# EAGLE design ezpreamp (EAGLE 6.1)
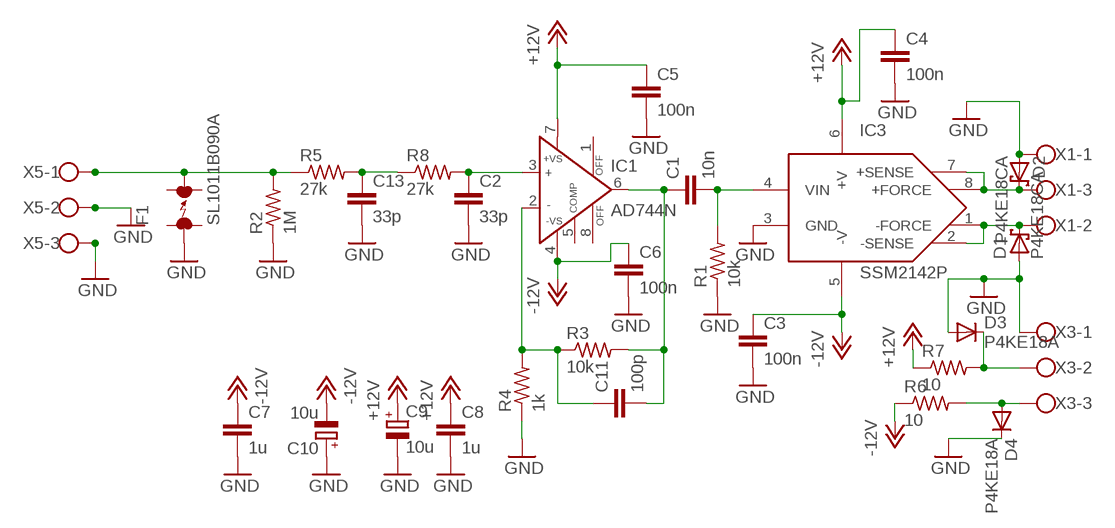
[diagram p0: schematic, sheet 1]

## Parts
C1  10n  C5/3  [C5B3]
C2  33p  C5/3  [C5B3]
C3  100n  C5/2.5  [C5B2.5]
C4  100n  C5/2.5  [C5B2.5]
C5  100n  C5/2.5  [C5B2.5]
C6  100n  C5/2.5  [C5B2.5]
C7  1u  C5/2.5  [C5B2.5]
C8  1u  C5/2.5  [C5B2.5]
C9  10u  CPOL-EUE5-10.5  [E5-10,5]
C10  10u  CPOL-EUE5-10.5  [E5-10,5]
C11  100p  C5/3  [C5B3]
C13  33p  C5/3  [C5B3]
D1  P4KE18CA  P4KEXX  [DO41-10]
D2  P4KE18CA  P4KEXX  [DO41-10]
D3  P4KE18A  1N4004  [DO41-10]
D4  P4KE18A  1N4004  [DO41-10]
F1  SL1011B090A  ARRESTER  [EPCOS_N81]
IC1  AD744N  [DIL08]
IC3  SSM2142P  [N-8]
R1  10k  R-US_0207/10  [0207/10]
R2  1M  R-US_0207/10  [0207/10]
R3  10k  R-US_0207/10  [0207/10]
R4  1k  R-US_0207/10  [0207/10]
R5  27k  R-US_0207/10  [0207/10]
R6  10  R-US_0207/10  [0207/10]
R7  10  R-US_0207/10  [0207/10]
R8  27k  R-US_0207/10  [0207/10]
X1  W237-103  [W237-103]
X3  W237-103  [W237-103]
X5  W237-103  [W237-103]

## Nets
+12V: C4.1 C5.1 C8.1 C9.+ IC1.7(+VS) IC3.6(+V) R7.1
-12V: C3.1 C6.1 C7.1 C10.- IC1.4(-VS) IC3.5(-V) R6.1
GND: C2.2 C3.2 C4.2 C5.2 C6.2 C7.2 C8.2 C9.- C10.+ C13.2 D1.A D2.A D3.A D4.C F1.1 IC3.3(GND) R1.1 R2.1 R4.1 X1.1 X3.1 X5.2 X5.3
N$1: C2.1 IC1.3(IN+) R8.2
N$2: C13.1 R5.2 R8.1
N$3: C1.2 IC3.4(VIN) R1.2
N$4: C1.1 C11.2 IC1.6(OUT) R3.2
N$5: F1.2 R2.2 R5.1 X5.1
N$6: D2.C IC3.7(+SENSE) IC3.8(+FORCE) X1.3
N$7: D1.C IC3.1(-FORCE) IC3.2(-SENSE) X1.2
N$8: C11.1 IC1.2(IN-) R3.1 R4.2
N$13: D4.A R6.2 X3.3
N$14: D3.C R7.2 X3.2
Unconnected: IC1.1(OFF) IC1.5(COMP) IC1.8(OFF)

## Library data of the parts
C1-C8 C11 C13 = capacitor-wima:C: CAPACITOR
C9 C10 = resistor:CPOL-EU: POLARIZED CAPACITOR, European symbol
D1 D2 = diode:P4KEXX: DIODE
D3 D4 = diode:1N4004: DIODE
F1 = discrete:ARRESTER: GASENTLADUNGSABLEITER 90V 10KA
IC1 = analog-devices:AD744: Precision, 500 ns Settling BiFET Op Amp Source: http://www.analog.com/static/imported-files/data_sheets/AD744.pdf; MF: ALTERA CORPORATION; MPN: AD744JNZ; OC_FARNELL: 1438362; OC_NEWARK: 59K4810
IC3 = JBB:SSM2142P
R1-R8 = rcl:R-US_: RESISTOR, American symbol
X1 X3 X5 = con-wago-500:W237-103: WAGO SCREW CLAMP; MPN: 237-103; OC_FARNELL: unknown; OC_NEWARK: 18M7116

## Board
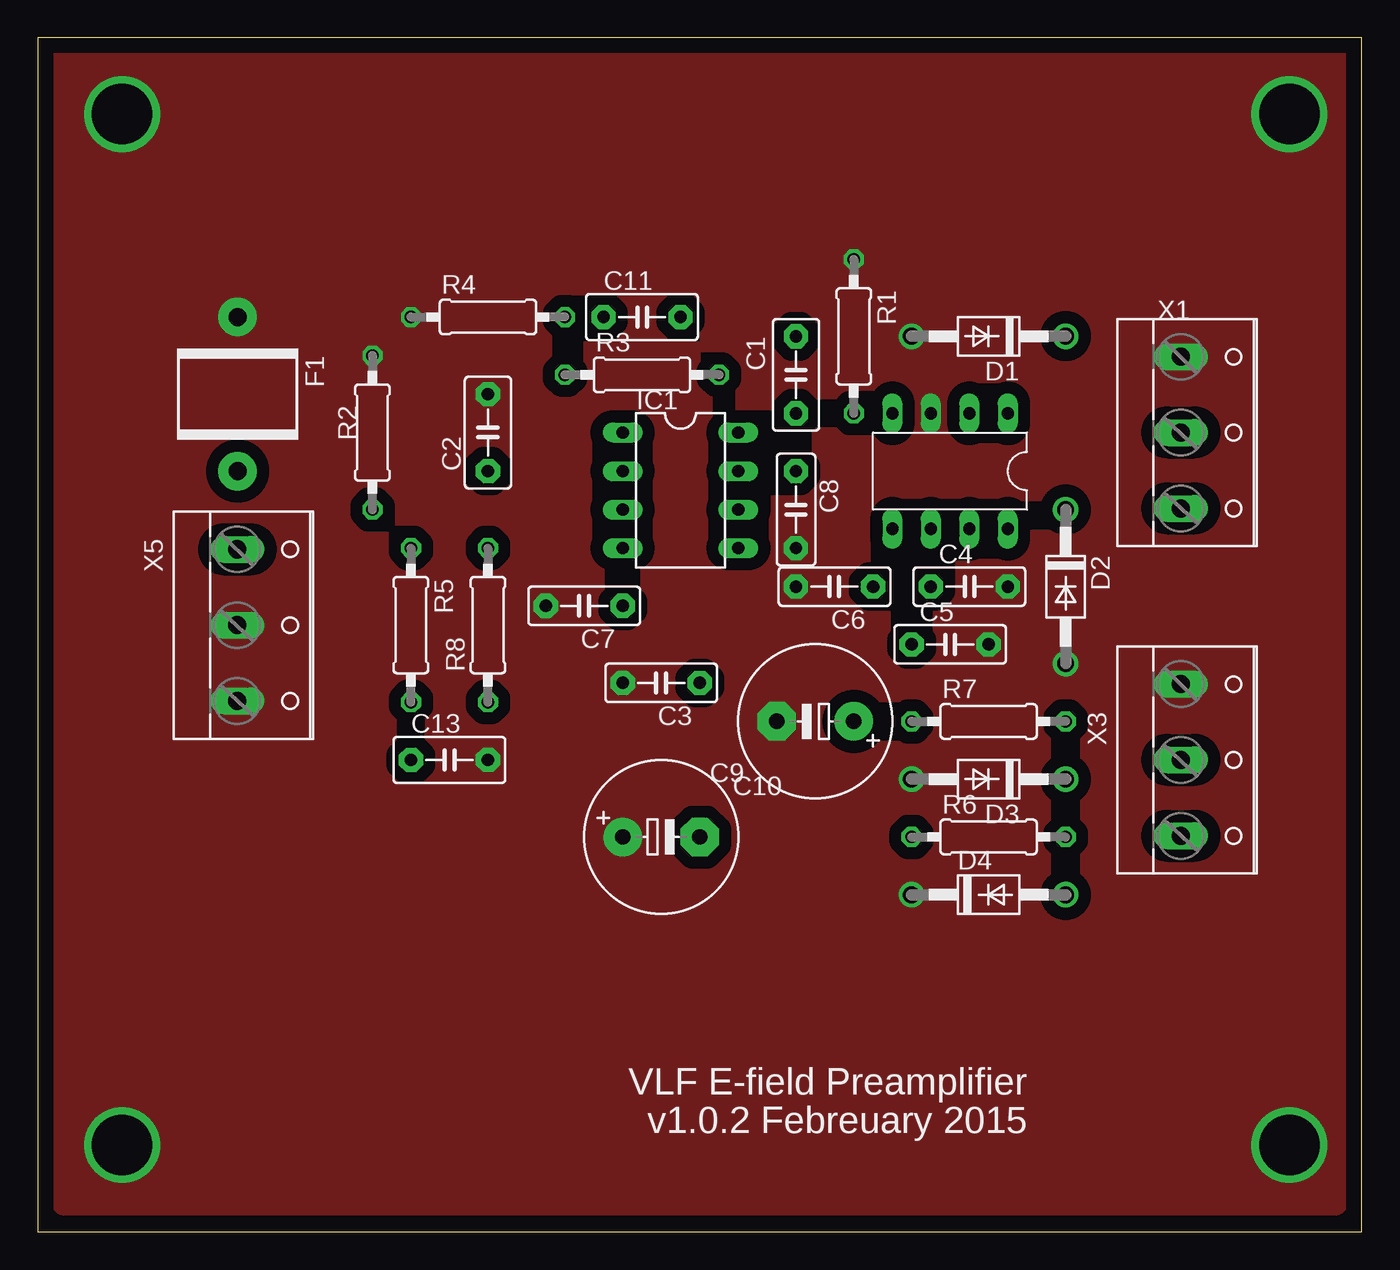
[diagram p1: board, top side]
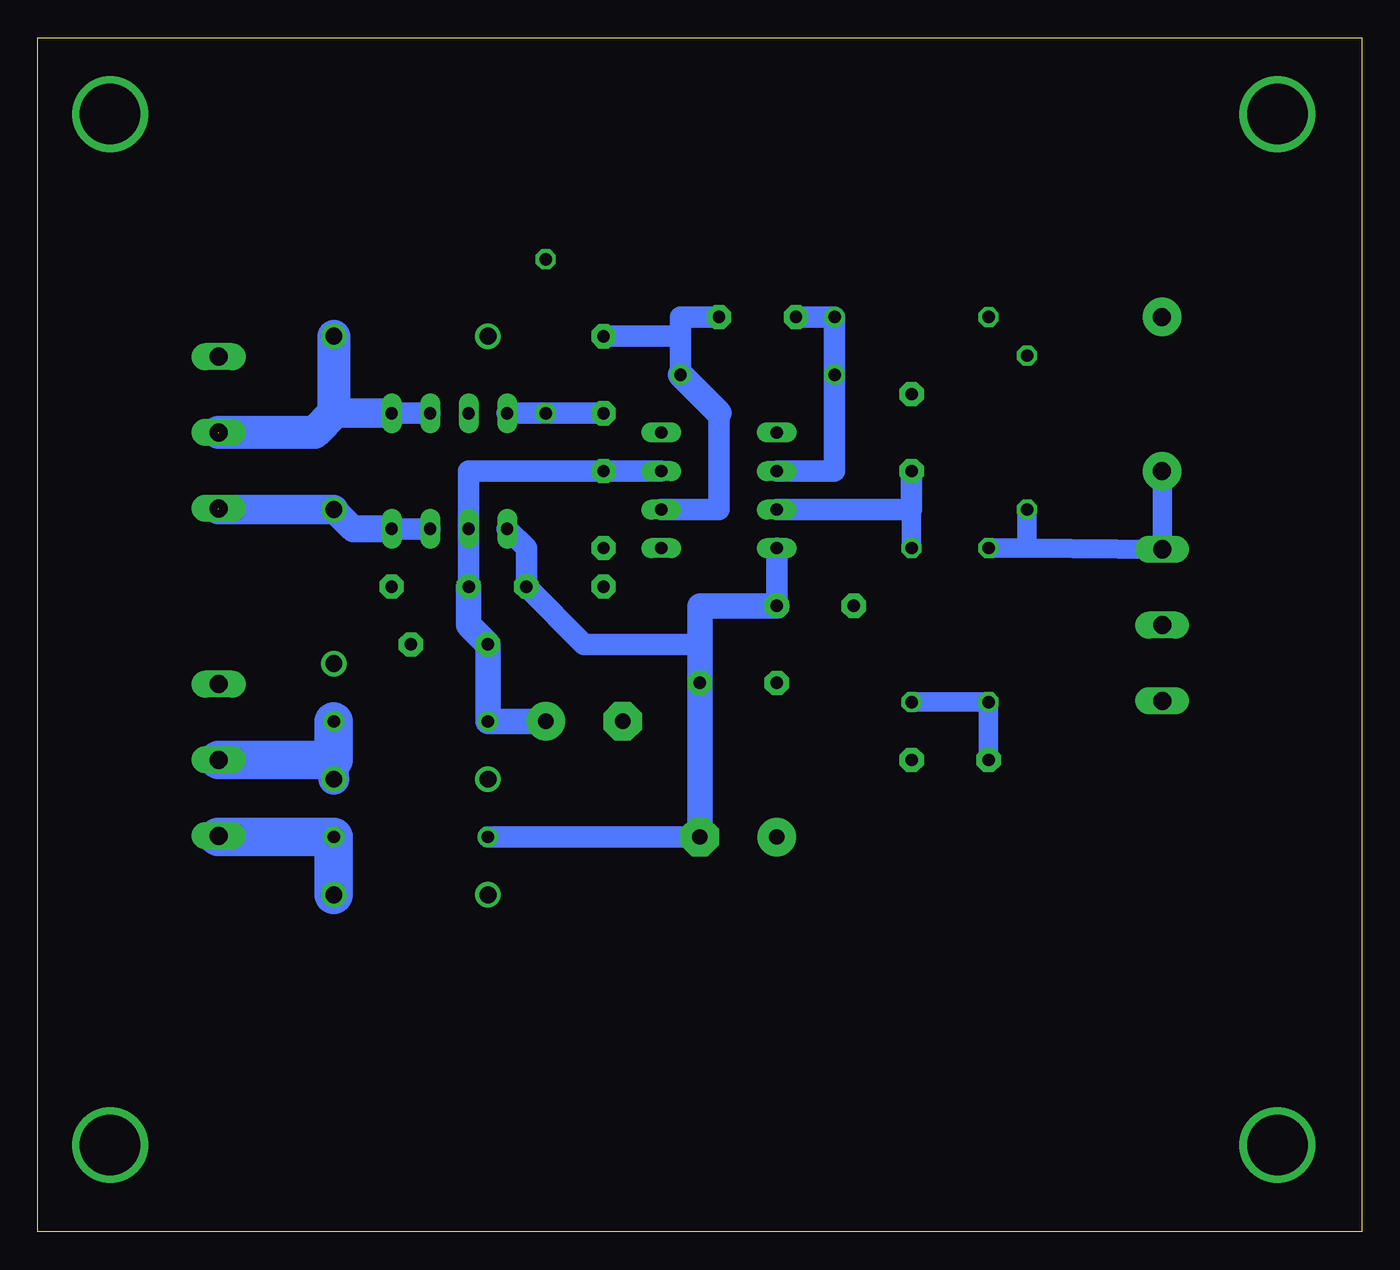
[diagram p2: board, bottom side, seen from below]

Size 87.3 x 78.73 mm. Coordinates in mm from the lower left corner, seen from the top.
Outline: 0,0 87.3,0 87.3,78.73 0,78.73 0,0
Copper layers (1*16): Top 0.035mm / dielectric 1.5mm / Bottom 0.035mm
Design rules: minimum track width 10mil, minimum drill 24mil, track to track 32mil, track to pad 34mil, pad to pad 32mil, via to via 32mil, smd to smd 16mil, copper to edge 40mil, drill to drill 8mil, minimum pad ring 10mil, minimum via ring 8mil, stop-mask expansion 4mil, vias tented up to drill 0mil, thermal gap 10mil

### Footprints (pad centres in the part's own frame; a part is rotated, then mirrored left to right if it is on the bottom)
C5B3 = drill 0.813 pad 1.6 octagon: 1 -2.54,0; 2 2.54,0
C5B2.5 = drill 0.813 pad 1.6 octagon: 1 -2.54,0; 2 2.54,0
E5-10,5 = drill 1.016 pad 2.54: + -2.54,0 | drill 1.016 pad 2.54 octagon: - 2.54,0
DO41-10 = drill 1.118: A 5.08,0; C -5.08,0
EPCOS_N81 = drill 1.2 pad 2.54: 1 -5.08,0; 2 5.08,0
DIL08 = drill 0.813 long: 1 -3.81,-3.81; 2 -1.27,-3.81; 3 1.27,-3.81; 4 3.81,-3.81; 5 3.81,3.81; 6 1.27,3.81; 7 -1.27,3.81; 8 -3.81,3.81
N-8 = drill 0.8 long: 1 0,0; 2 2.54,0; 3 5.08,0; 4 7.62,0; 5 7.62,7.62; 6 5.08,7.62; 7 2.54,7.62; 8 0,7.62
0207/10 = drill 0.813 octagon: 1 -5.08,0; 2 5.08,0
W237-103 = drill 1.194 long: 1 -5,-1.29; 2 0,-1.29; 3 5,-1.29

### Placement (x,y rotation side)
C1  50,56.51 270 top
C2  29.68,52.7 90 top
C3  41.11,36.19 180 top
C4  61.43,42.54 0 top
C5  60.16,38.73 0 top
C6  52.54,42.54 180 top
C7  36.03,41.27 180 top
C8  50,47.62 270 top
C9  51.27,33.65 180 top
C10  41.11,26.03 0 top
C11  39.84,60.32 0 top
C13  27.14,31.11 0 top
D1  62.7,59.05 180 top
D2  67.78,42.54 270 top
D3  62.7,29.84 180 top
D4  62.7,22.22 0 top
F1  13.17,55.24 270 top
IC1  42.38,48.89 270 top
IC3  63.97,53.97 180 top
R1  53.81,59.05 270 top
R2  22.06,52.7 270 top
R3  39.84,56.51 0 top
R4  29.68,60.32 0 top
R5  24.6,40 270 top
R6  62.7,26.03 0 top
R7  62.7,33.65 0 top
R8  29.68,40 90 top
X1  76.67,52.7 270 top
X3  76.67,31.11 270 top
X5  14.44,40 270 top

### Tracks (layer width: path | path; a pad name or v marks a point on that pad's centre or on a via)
+12V
  Bottom 1.422: C4.1 IC3.6 58.89,50.16 C8.1 IC1.7
  Bottom 1.676: C9.+ R7.1 C5.1 58.89,40 C4.1
-12V
  Bottom 1.422: 43.65,38.73 51.27,38.73 C6.1 55.08,45.08 IC3.5 | IC1.4 C7.1 | R6.1 C10.-
  Bottom 1.676: C7.1 43.65,41.27 43.65,38.73 C10.- C3.1
GND  (via drill 3.99)
  other vias: 5.55,5.71 5.55,73.71 82.54,73.71 82.54,5.71
  pour Top (no thermals): 1.74,78.1 1.74,1.9 85.56,1.9 85.56,78.1
N$1
  Bottom 1.27: R8.2 29.68,47.62
  Bottom 1.422: C2.1 29.68,47.62 IC1.3
N$2
  Bottom 1.27: C13.1 R5.2 R8.1
N$3
  Bottom 1.422: C1.2 R1.2 IC3.4
N$4
  Bottom 1.422: C11.2 44.92,60.32 44.92,59.05 | 44.92,59.05 R3.2 | 42.38,53.97 42.38,47.62 IC1.6 | C1.1 44.92,59.05
  Bottom 1.676: 42.38,53.97 R3.2
N$5
  Bottom 0.406: F1.2 13.15,50.16
  Bottom 1.27: 13.15,50.16 X5.1 22.06,45.08 | R5.1 22.06,45.08 | R2.2 22.06,45.08
N$6  (1 unrouted)
  Bottom 1.422: IC3.7 IC3.8
  Bottom 1.778: IC3.8 66.51,46.35 D2.C
  Bottom 1.93: D2.C 75.4,47.62
N$7  (1 unrouted)
  Bottom 1.422: IC3.2 IC3.1
  Bottom 1.93: IC3.1 67.78,53.97
  Bottom 2.184: D1.C 67.78,53.97 69.05,52.7 75.4,52.7
N$8
  Bottom 1.422: IC1.2 34.76,50.16 R4.2 | R4.2 C11.1 | R4.2 R3.1
N$13
  Bottom 1.422: 75.4,26.03 75.4,26.11 X3.3
  Bottom 2.54: 75.4,26.03 R6.2 D4.A
N$14
  Bottom 1.422: X3.2 75.4,31.11
  Bottom 2.032: D3.C R7.2
  Bottom 2.54: R7.2 67.78,31.11 X3.2

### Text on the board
tNames: VLF E-field Preamplifier | v1.0.2 Febreuary 2015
